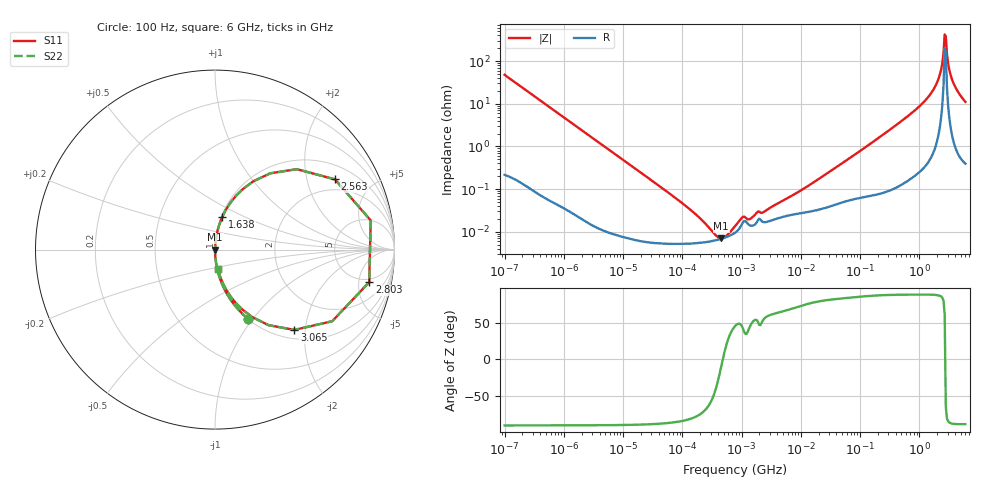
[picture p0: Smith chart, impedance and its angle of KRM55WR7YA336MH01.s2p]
!Murata Part Number: KRM55WR7YA336MH01
!These Parameters are Measured in Series Mode Connection
!Data Generated on Jan 08, 2026
!  o--ll--o
!Port1  Port2
!  o------o
!Operation Temp=25[degC], DC Bias Voltage=0[V]
!Freq. Start=100[Hz] Stop=6[GHz] 401[Steps]
# Hz S RI R 50
!Freq.(Hz) S11(Real) S11(Imag) S21(Real) S21(Imag) S12(Real) S12(Imag) S22(Real) S22(Imag)
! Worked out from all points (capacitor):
!   401 points, 100 Hz to 6 GHz, reference 50 ohm
!   read as one part in series: C = 33.3 uF near 109 Hz
!   lowest |Z| = 6.99 mohm at 452.6 kHz (marker M1)
!   series resonance near 480.9 kHz, so ESL is about 3.3 nH
!   S11 on the Smith chart (normalised r, x): 100 Hz: 1.00, -0.95; 1.638 GHz: 1.01, +0.38; 2.563 GHz: 1.52, +2.97; 2.803 GHz: 4.33, -6.88; 3.065 GHz: 1.18, -1.75; 6 GHz: 1.01, -0.22
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100  0.1865 -0.3872  0.8135 0.3872  0.8135 0.3872  0.1865 -0.3872
383  0.0161 -0.123  0.9839 0.123  0.9839 0.123  0.0161 -0.123
2008  0.000775 -0.024  0.9992 0.024  0.9992 0.024  0.000775 -0.024
40335  5.51e-05 -0.0012  0.9999 0.0012  0.9999 0.0012  5.51e-05 -0.0012
316350  6.08e-05 -8.5e-05  0.9999 8.5e-05  0.9999 8.5e-05  6.08e-05 -8.5e-05
452617  6.89e-05 -1.17e-05  0.9999 1.17e-05  0.9999 1.17e-05  6.89e-05 -1.17e-05
619225  8.05e-05 4.92e-05  0.9999 -4.92e-05  0.9999 -4.92e-05  8.05e-05 4.92e-05
774597  9.51e-05 9.62e-05  0.9999 -9.62e-05  0.9999 -9.62e-05  9.51e-05 9.62e-05
1013323  0.000151 0.000153  0.9998 -0.000153  0.9998 -0.000153  0.000151 0.000153
2372521  0.000168 0.000239  0.9998 -0.000239  0.9998 -0.000239  0.000168 0.000239
1.555665e7  0.000307 0.00134  0.9997 -0.00134  0.9997 -0.00134  0.000307 0.00134
3.124326e8  0.0015 0.0241  0.9985 -0.0241  0.9985 -0.0241  0.0015 0.0241
9.150511e8  0.00818 0.0767  0.9918 -0.0767  0.9918 -0.0767  0.00818 0.0767
1.637704e9  0.0402 0.1812  0.9598 -0.1812  0.9598 -0.1812  0.0402 0.1812
2.142435e9  0.156 0.338  0.844 -0.338  0.844 -0.338  0.156 0.338
2.34314e9  0.3084 0.4251  0.6916 -0.4251  0.6916 -0.4251  0.3084 0.4251
2.562649e9  0.6684 0.3913  0.3316 -0.3913  0.3316 -0.3913  0.6684 0.3913
2.802721e9  0.8593 -0.1816  0.1407 0.1816  0.1407 0.1816  0.8593 -0.1816
3.065283e9  0.4426 -0.4474  0.5574 0.4474  0.5574 0.4474  0.4426 -0.4474
3.205649e9  0.2982 -0.4209  0.7018 0.4209  0.7018 0.4209  0.2982 -0.4209
3.666503e9  0.1123 -0.2935  0.8877 0.2935  0.8877 0.2935  0.1123 -0.2935
6e9  0.0159 -0.1085  0.9841 0.1085  0.9841 0.1085  0.0159 -0.1085
